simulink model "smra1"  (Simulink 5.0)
settings: Solver=ode4  StartTime=0.0  StopTime=10.0  RelTol=1e-3
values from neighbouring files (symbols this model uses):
  B = 8    [smra1_1dat.m]
  k = 80    [smra1_1dat.m]
  m = 2    [smra1_1dat.m]
  v0 = 0    [smra1_1dat.m]
  x0 = 10    [smra1_1dat.m]

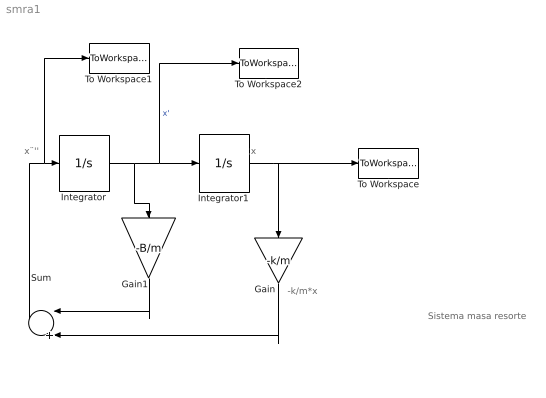
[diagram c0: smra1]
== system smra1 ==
  note: x¨''
  note: x
  note: Sistema masa resorte
  note: -k/m*x
  Gain : Gain  Orientation=down  Gain=-k/m
  Gain1 : Gain  Orientation=down  Gain=-B/m
  Integrator : Integrator  InitialCondition=v0
  Integrator1 : Integrator  InitialCondition=x0
  Sum : Sum  Orientation=left  Inputs=|++
  To Workspace : ToWorkspace  VariableName=pos  SampleTime=-1  SaveFormat=Array
  To Workspace1 : ToWorkspace  VariableName=ace  SampleTime=-1  SaveFormat=Array
  To Workspace2 : ToWorkspace  VariableName=vel  SampleTime=-1  SaveFormat=Array
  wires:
  Integrator/1 -> Integrator1/1, To Workspace2/1, Gain1/1  "x'"
  Integrator1/1 -> Gain/1, To Workspace/1
  Gain1/1 -> Sum/1
  Gain/1 -> Sum/2
  Sum/1 -> Integrator/1, To Workspace1/1
